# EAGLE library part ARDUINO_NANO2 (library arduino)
Arduino Nano2 Auto generated by modulcreator.ulp \;
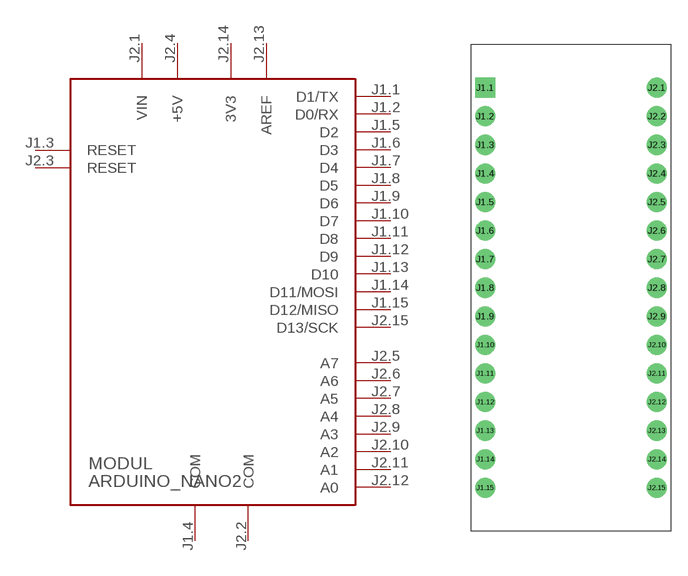
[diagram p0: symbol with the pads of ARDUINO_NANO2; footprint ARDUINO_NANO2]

Designator prefix MODUL

## ARDUINO_NANO2 (ANZAHL: 2; MODUL: TRUE; STECKX0: -76200; STECKX1: 76200; STECKY0: 177800; STECKY1: 177800)  [ARDUINO_NANO2]
J1.1  D1/TX
J1.2  D0/RX
J1.3  RESET
J1.4  COM  pwr
J1.5  D2
J1.6  D3
J1.7  D4
J1.8  D5
J1.9  D6
J1.10  D7
J1.11  D8
J1.12  D9
J1.13  D10
J1.14  D11/MOSI
J1.15  D12/MISO
J2.1  VIN  pwr
J2.2  COM  pwr
J2.3  RESET
J2.4  +5V  pwr
J2.5  A7
J2.6  A6
J2.7  A5
J2.8  A4
J2.9  A3
J2.10  A2
J2.11  A1
J2.12  A0
J2.13  AREF  pwr
J2.14  3V3  pwr
J2.15  D13/SCK

## Footprint ARDUINO_NANO2 (pad centres in mm)
Arduino Nano2 Auto generated by modulcreator.ulp \;
drill 0.914 pad 1.778 square: J1.1 -7.62,17.78
drill 0.914 pad 1.778: J1.2 -7.62,15.24; J1.3 -7.62,12.7; J1.4 -7.62,10.16; J1.5 -7.62,7.62; J1.6 -7.62,5.08; J1.7 -7.62,2.54; J1.8 -7.62,0; J1.9 -7.62,-2.54; J1.10 -7.62,-5.08; J1.11 -7.62,-7.62; J1.12 -7.62,-10.16; J1.13 -7.62,-12.7; J1.14 -7.62,-15.24; J1.15 -7.62,-17.78; J2.1 7.62,17.78; J2.2 7.62,15.24; J2.3 7.62,12.7; J2.4 7.62,10.16; J2.5 7.62,7.62; J2.6 7.62,5.08; J2.7 7.62,2.54; J2.8 7.62,0; J2.9 7.62,-2.54; J2.10 7.62,-5.08; J2.11 7.62,-7.62; J2.12 7.62,-10.16; J2.13 7.62,-12.7; J2.14 7.62,-15.24; J2.15 7.62,-17.78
